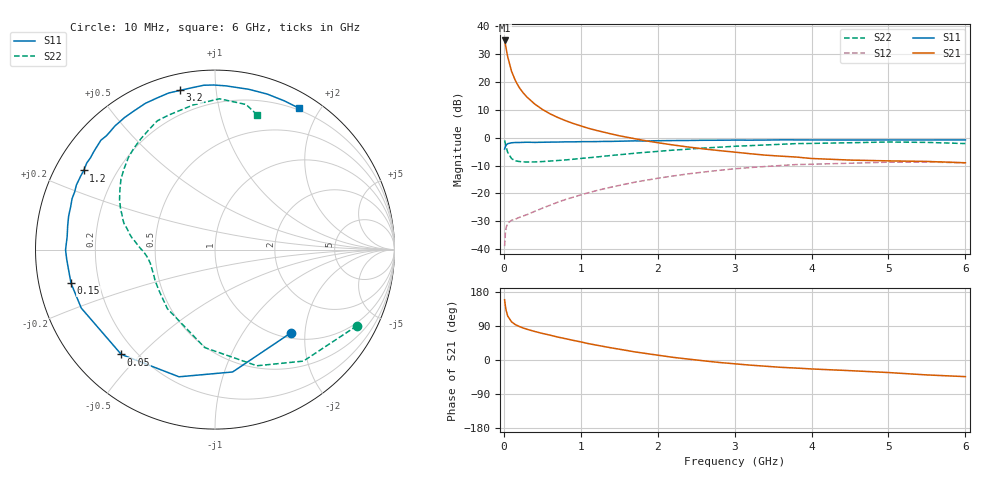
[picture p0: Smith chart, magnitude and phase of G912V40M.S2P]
! SIEMENS Small Signal Semiconductors
! BFG235
! Si NPN RF Bipolar Junction Transistor in SOT223
! VCE = 12 V  IC = 40 mA
! Common Emitter S-Parameters:  July  1994
# GHz  S  MA  R  50
!  f  S11  S21  S12  S22
! GHz  MAG  ANG  MAG  ANG  MAG  ANG  MAG  ANG
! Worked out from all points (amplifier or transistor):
!   40 points, 10 MHz to 6 GHz, reference 50 ohm
!   highest |S21| = 35.0 dB at 10 MHz (marker M1)
!   |S21| within 3 dB of that: start of sweep to 30.77 MHz
!   unconditionally stable (mu >= 1): 516.9 MHz to 1.29 GHz
!   at 200 MHz: K = 0.59, MSG = 23.3 dB, |S12| = -28.6 dB
!   at 1.5 GHz: K = 0.97, MSG = 8.9 dB, |S12| = -17.1 dB
!   at 6 GHz: K = 0.94, MSG = 0.0 dB, |S12| = -9.0 dB
!   S11 on the Smith chart (normalised r, x): 10 MHz: 1.11, -1.70; 50 MHz: 0.15, -0.44; 150 MHz: 0.10, -0.11; 1.2 GHz: 0.08, +0.28; 3.2 GHz: 0.08, +0.80; 6 GHz: 0.18, +1.75
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0.01  0.6281 -47.4  56.08 159.0  0.0113 70.0  0.8977 -28.2
0.02  0.6888 -81.8  47.77 142.6  0.0192 55.3  0.7928 -51.6
0.03  0.7365 -105.8  40.23 130.6  0.0245 45.6  0.6879 -70.2
0.05  0.7834 -131.8  28.58 116.1  0.0292 35.0  0.5488 -96.0
0.1  0.8133 -156.4  15.7 100.7  0.0329 28.3  0.4227 -128.9
0.15  0.8237 -166.8  10.65 93.3  0.0346 29.7  0.3859 -144.4
0.2  0.8236 -172.2  8.007 88.5  0.0371 32.2  0.375 -153.2
0.25  0.8283 -176.5  6.449 84.5  0.0393 35.5  0.3686 -158.7
0.3  0.8326 -179.9  5.4 81.3  0.0416 38.6  0.3675 -162.9
0.4  0.8269 174.9  4.059 75.4  0.0477 44.0  0.3685 -168.0
0.5  0.8316 170.7  3.243 70.2  0.0542 48.0  0.3741 -171.5
0.6  0.8364 167.1  2.7 65.6  0.0615 50.5  0.382 -174.4
0.7  0.839 163.4  2.323 60.6  0.0696 52.4  0.3909 -176.7
0.9  0.8455 157.5  1.813 51.9  0.0855 54.1  0.4119 179.6
1.1  0.8532 151.2  1.481 43.2  0.1031 54.1  0.4381 175.6
1.2  0.854 148.9  1.362 39.4  0.1121 53.9  0.4509 173.8
1.7  0.8806 136.2  0.964 21.5  0.159 48.8  0.5281 163.9
2.2  0.8918 124.4  0.743 7.0  0.2061 40.6  0.6002 152.4
3.2  0.908 102.3  0.518 -13.5  0.2917 20.4  0.723 128.8
4.5  0.9128 78.1  0.398 -28.1  0.3494 -6.8  0.8149 98.6
5.5  0.9143 65.0  0.376 -39.4  0.367 -25.9  0.8267 77.9
6  0.9166 59.2  0.356 -43.9  0.3549 -32.8  0.7879 72.8
